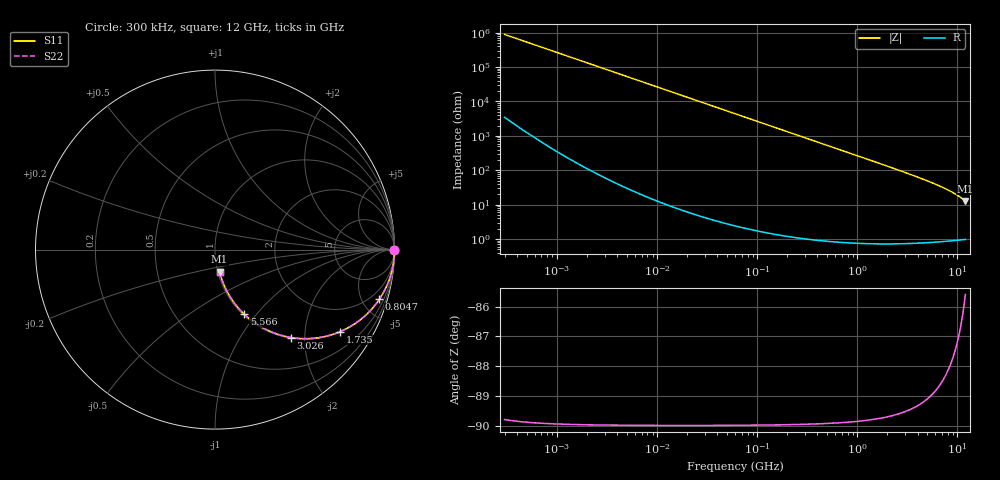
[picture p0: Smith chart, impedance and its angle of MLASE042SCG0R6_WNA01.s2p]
! MLASE042SCG0R6_WNA01  S-PARAMETER MODEL  ( General Type )
! Model Generated by TAIYO YUDEN Corporation (http://www.ty-top.com)
! Version 1.0
! TAIYO YUDEN Control No. 130801
! Copyright(c) 2013 TAIYO YUDEN CO.,LTD. All Rights Reserved.
! Product Description (link to TY-COMPAS)
! https://ds.yuden.co.jp/TYCOMPAS/or/detail?pn=MLASE042SCG0R6AWNA01&u=M
! Products Name : Multilayer Ceramic Capacitors
! Characteristics :
!  Capacitance : 0.6 pF , Rated Voltage : 16V , TCC : CG / C0G
!  Case Size : 0.4 x 0.2 / 0.016 x 0.008 [mm/inch] , Thickness : 0.2 / 0.008 [mm/inch]
!  (Conditions: Temperature = 25 degC , DC Bias Current/Voltage = 0A / 0V)
! External Node Assignments :
!  1  o---| |---o  2
! GND o---------o GND
! Frequency Range : 0.3MHz  -  12000MHz  [ 401 STEP ]
# MHz S RI R 50
! Freq[MHz].  S11 Real  S11 Imag  S21 Real  S21 Imag  S12 Real  S12 Imag  S22 Real  S22 Imag
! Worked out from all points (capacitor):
!   401 points, 300 kHz to 12 GHz, reference 50 ohm
!   read as one part in series: C = 598 fF near 316.3 kHz
!   lowest |Z| = 12.7 ohm at 12 GHz (marker M1)
!   S11 on the Smith chart (normalised r, x): 300 kHz: open; 804.7 MHz: 1.02, -6.60; 1.735 GHz: 1.01, -3.04; 3.026 GHz: 1.01, -1.71; 5.566 GHz: 1.02, -0.87; 12 GHz: 1.02, -0.25
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0.3  1 -0.000113  4.52e-07 0.000113  4.52e-07 0.000113  1 -0.000113
0.316324  1 -0.000119  4.52e-07 0.000119  4.52e-07 0.000119  1 -0.000119
1.769972  1 -0.000665  1.04e-06 0.000665  1.04e-06 0.000665  1 -0.000665
10.44266  1 -0.00392  1.73e-05 0.00392  1.73e-05 0.00392  1 -0.00392
60  0.9995 -0.0225  0.000521 0.0225  0.000521 0.0225  0.9995 -0.0225
164.1901  0.9962 -0.0615  0.00384 0.0615  0.00384 0.0615  0.9962 -0.0615
353.9943  0.9824 -0.1307  0.0176 0.1307  0.0176 0.1307  0.9824 -0.1307
555.3718  0.9579 -0.2  0.0421 0.2  0.0421 0.2  0.9579 -0.2
804.7407  0.9153 -0.2772  0.0847 0.2772  0.0847 0.2772  0.9153 -0.2772
1197.383  0.8296 -0.3743  0.1704 0.3743  0.1704 0.3743  0.8296 -0.3743
1441.349  0.77 -0.4188  0.23 0.4188  0.23 0.4188  0.77 -0.4188
1735.023  0.697 -0.4572  0.303 0.4572  0.303 0.4572  0.697 -0.4572
2088.533  0.612 -0.4844  0.388 0.4844  0.388 0.4844  0.612 -0.4844
2514.07  0.5188 -0.4962  0.4812 0.4962  0.4812 0.4962  0.5188 -0.4962
3026.31  0.4232 -0.4898  0.5768 0.4898  0.5768 0.4898  0.4232 -0.4898
3944.255  0.295 -0.4502  0.705 0.4502  0.705 0.4502  0.295 -0.4502
5565.855  0.1632 -0.3604  0.8368 0.3604  0.8368 0.3604  0.1632 -0.3604
6879.757  0.1055 -0.2949  0.8945 0.2949  0.8945 0.2949  0.1055 -0.2949
8503.825  0.0643 -0.228  0.9357 0.228  0.9357 0.228  0.0643 -0.228
9708.23  0.0456 -0.1868  0.9544 0.1868  0.9544 0.1868  0.0456 -0.1868
11380.75  0.0293 -0.1385  0.9707 0.1385  0.9707 0.1385  0.0293 -0.1385
12000  0.0251 -0.1227  0.9749 0.1227  0.9749 0.1227  0.0251 -0.1227
